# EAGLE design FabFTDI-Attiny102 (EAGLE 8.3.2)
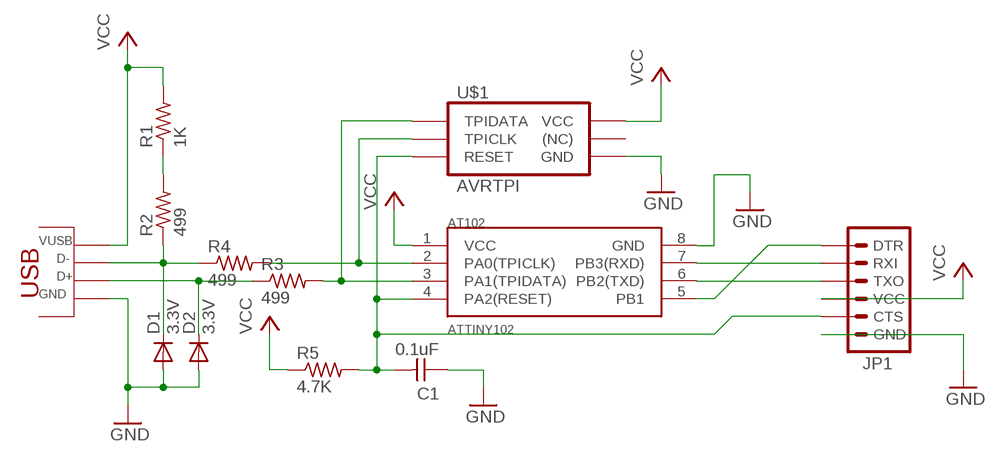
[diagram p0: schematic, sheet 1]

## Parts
C1  0.1uF  UNPOLARIZED_CAPACITOR1206  [1206]
D1  3.3V  DIODESOD123  [SOD123]
D2  3.3V  DIODESOD123  [SOD123]
IC1  ATTINY102  ATTINY102/104  [SOIC8]
JP1  FTDI_CONNECTORSMD  [1X06-SMD]
R1  1K  RESISTOR1206  [1206]
R2  499  RESISTOR1206  [1206]
R3  499  RESISTOR1206  [1206]
R4  499  RESISTOR1206  [1206]
R5  4.7K  RESISTOR1206  [1206]
U$1  AVRTPI  AVRTPISMD  [2X03SMD]
U$3  USB_PCB  [USB_PCB]

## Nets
DELTE: D2.CATHODE(C) R3.1 U$3.D+
GND: C1.1 D1.ANODE(A) D2.ANODE(A) IC1.8(GND) JP1.6(GND) U$1.6(GND) U$3.GND
N$1: R1.1 R2.2
N$2: IC1.7(PB3(RXD)) JP1.2(RXI)
N$3: IC1.6(PB2(TXD)) JP1.3(TXO)
N$4: IC1.3(PA1(TPIDATA)) R3.2 U$1.1(TPIDATA)
N$5: C1.2 IC1.4(PA2(RESET)) JP1.5(CTS) R5.2 U$1.5(RESET)
N$6: IC1.5(PB1) JP1.1(DTR)
N$11: D1.CATHODE(C) R2.1 R4.1 U$3.D-
N$12: IC1.2(PA0(TPICLK)) R4.2 U$1.3(TPICLK)
VCC: IC1.1(VCC) JP1.4(VCC) R1.2 R5.1 U$1.2(VCC) U$3.5V(VUSB)
Unconnected: U$1.4((NC))

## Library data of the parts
C1 = fabPatil:UNPOLARIZED_CAPACITOR: unpolarized_capacitor
D1 D2 = fabPatil:DIODE: DIODE
IC1 = fabPatil:ATTINY102/104: ATTINY102/104 Device for ATTINY102/104
JP1 = fabPatil:FTDI_CONNECTOR: FTDI connector smd
R1-R5 = fabPatil:RESISTOR
U$1 = fabPatil:AVRTPI: ATMEL-ICE TPI Connector SMD This is a TPI programming connector to program Atiny102/104 micro-controllers prashant.patil@cba.mit.edu
U$3 = fabPatil:USB_PCB

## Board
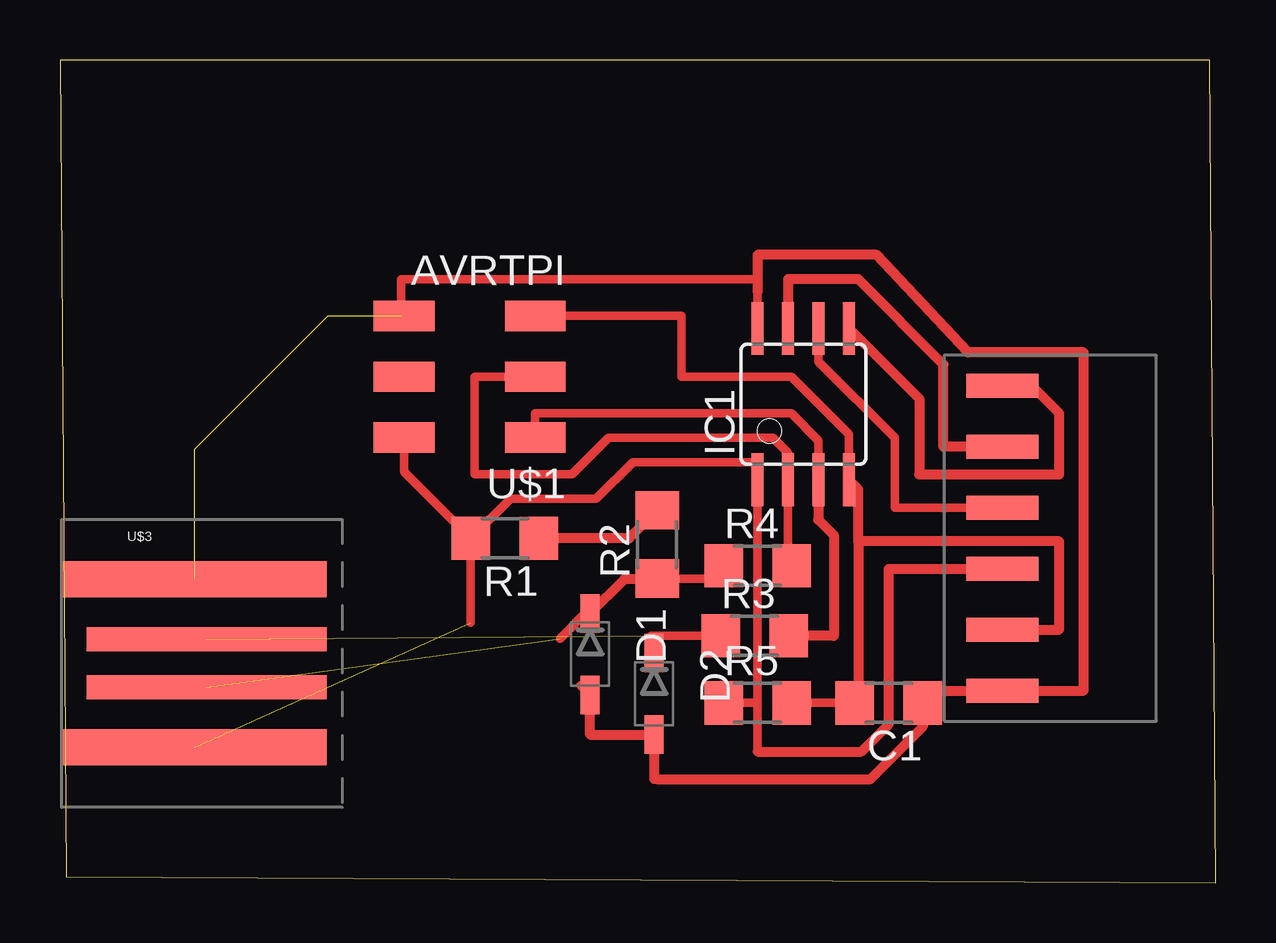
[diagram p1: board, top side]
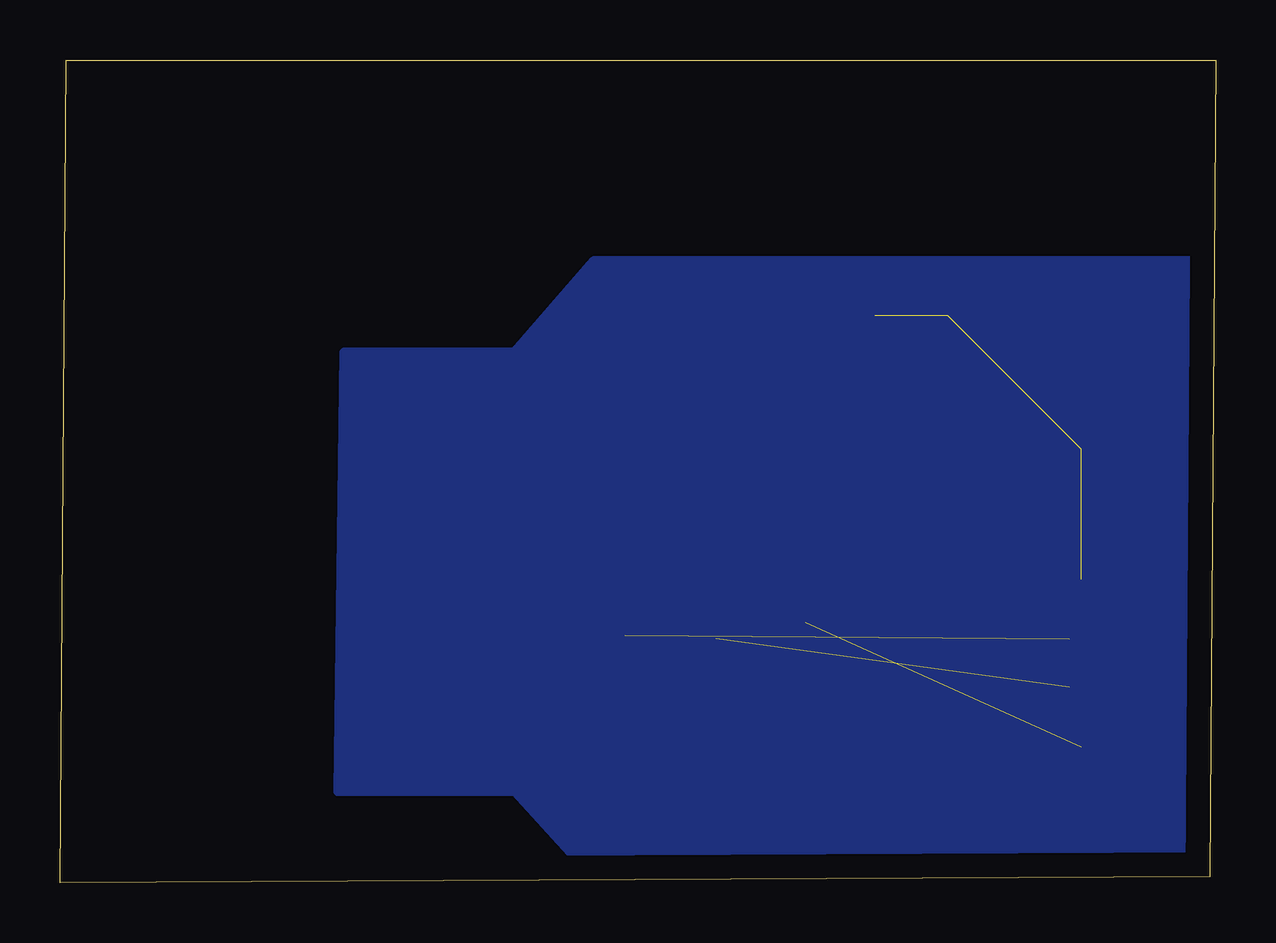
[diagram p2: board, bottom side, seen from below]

Size 48.18 x 34.28 mm. Coordinates in mm from the lower left corner, seen from the top.
Outline: 0.25,0.25 48.18,0 47.93,34.28 0,34.28 0.25,0.25
Copper layers (1*16): Top 0.035mm / dielectric 1.5mm / Bottom 0.035mm
Design rules "default": minimum track width 6mil, minimum drill 0.35mm, track to track 6mil, track to pad 6mil, pad to pad 6mil, via to via 6mil, smd to smd 6mil, copper to edge 40mil, drill to drill 6mil, minimum pad ring 10mil, minimum via ring 8mil, stop-mask expansion 4mil, vias tented up to drill 0mil, thermal gap 10mil

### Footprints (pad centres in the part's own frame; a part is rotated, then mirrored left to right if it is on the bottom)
1206 = smd 1.6 x 1.803: 1 -1.422,0; 2 1.422,0
SOD123 = smd 1.6 x 0.8: ANODE 1.7,0; CATHODE -1.7,0
SOIC8 = smd 0.5 x 2.2: 1 -1.905,-3.154; 2 -0.645,-3.154; 3 0.625,-3.154; 4 1.895,-3.154; 5 1.905,3.154; 6 0.635,3.154; 7 -0.635,3.154; 8 -1.905,3.154
1X06-SMD = smd 1 x 3: 1 -6.35,-1.35; 2 -3.81,-1.35; 3 -1.27,-1.35; 4 1.27,-1.35; 5 3.81,-1.35; 6 6.35,-1.35
2X03SMD = smd 2.54 x 1.27: 1 -2.54,2.54; 2 2.92,2.54; 3 -2.54,0; 4 2.92,0; 5 -2.54,-2.54; 6 2.92,-2.54
USB_PCB = smd 11 x 1.5: 5V 1.55,-3.5; GND 1.55,3.5 | smd 10 x 1: D+ 2.05,1; D- 2.05,-1

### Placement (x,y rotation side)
C1  34.54,7.49 180 top
D1  22.1,9.53 270 top
D2  24.77,7.87 270 top
IC1  30.99,19.94 0 top
JP1  40.64,14.35 270 top
R1  18.54,14.35 180 top
R2  24.89,14.1 90 top
R3  28.96,10.29 0 top
R4  29.08,13.21 0 top
R5  29.08,7.49 0 top
U$1  17.27,21.08 180 top
U$3  4.06,9.14 0 top

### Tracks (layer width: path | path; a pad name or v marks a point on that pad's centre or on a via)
DELTE  (1 unrouted)
  Top 0.356: 24.72,9.53 24.64,9.53 24.64,10.29 R3.1
  Top 0.406: 24.72,9.53 arc90 D2.CATHODE
GND  (3 unrouted)
  Top 0.356: D1.ANODE 21.7,8.22 | IC1.8 29.08,24.64 29.08,25.15 14.22,25.15 14.22,23.62 U$1.6
  Top 0.406: D1.ANODE 22.1,6.17 D2.ANODE 24.77,4.45 24.89,4.32 | 36.47,8 C1.1 | 29.08,24.64 29.08,26.16 34.04,26.16 37.85,22.1 42.67,22.1 42.67,8 JP1.6 35.97,8 C1.1 | C1.1 36.07,7.49 | C1.1 35.97,6.5 33.78,4.32 24.89,4.32 | 24.89,4.32 24.77,4.32
N$1
  Top 0.406: R2.2 23.72,14.35 R1.1
N$2
  Top 0.406: IC1.7 30.35,25.15 33.27,25.15 36.83,21.59 36.83,18.16 JP1.2
N$3
  Top 0.356: JP1.3 34.8,15.62 34.8,18.54 31.62,21.72 IC1.6
N$4
  Top 0.356: U$1.1 19.81,19.56 30.48,19.56 31.61,18.43 IC1.3
  Top 0.406: R3.2 32.26,10.29 32.26,14.48 31.61,15.12 IC1.3
N$5
  Top 0.356: U$1.5 25.91,23.62 25.91,21.08 30.48,21.08 32.88,18.68 IC1.4 | R5.2 C1.2
  Top 0.406: C1.2 33.27,7.75 33.27,14.22 | 33.27,14.22 33.27,16.39 IC1.4 | JP1.5 41.66,10.54 41.66,14.22 33.27,14.22
N$6
  Top 0.406: JP1.1 39.42,20.57 40.64,20.57 41.66,19.56 41.66,17.02 35.81,17.02 35.81,20.17 IC1.5
N$7
  pour Bottom: 26.67,1.02 29.21,3.81 36.58,3.81 36.32,22.1 29.21,22.1 25.91,25.91 1.02,25.91 1.27,1.02
N$11  (1 unrouted)
  Top 0.356: D1.CATHODE 22.1,11.43 20.84,10.18 | 24.89,12.7 R2.1 25.15,12.68 27.13,12.68 R4.1
  Top 0.406: 22.1,11.18 D1.CATHODE 23.55,12.68 25.15,12.68
N$12
  Top 0.356: U$1.3 17.27,21.08 17.27,17.02 21.34,17.02 22.86,18.54 29.72,18.54 30.34,17.92 IC1.2 30.34,13.21 R4.2
VCC  (1 unrouted)
  Top 0.356: R1.2 17.12,10.83 | R1.2 14.35,17.12 U$1.2 | R1.2 18.77,16 22.35,16 23.88,17.53 29.08,17.53 IC1.1 29.08,7.49 | 29.08,7.49 R5.1 | 29.08,7.49 29.08,5.46
  Top 0.406: JP1.4 34.54,13.08 34.54,6.6 33.4,5.46 29.08,5.46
